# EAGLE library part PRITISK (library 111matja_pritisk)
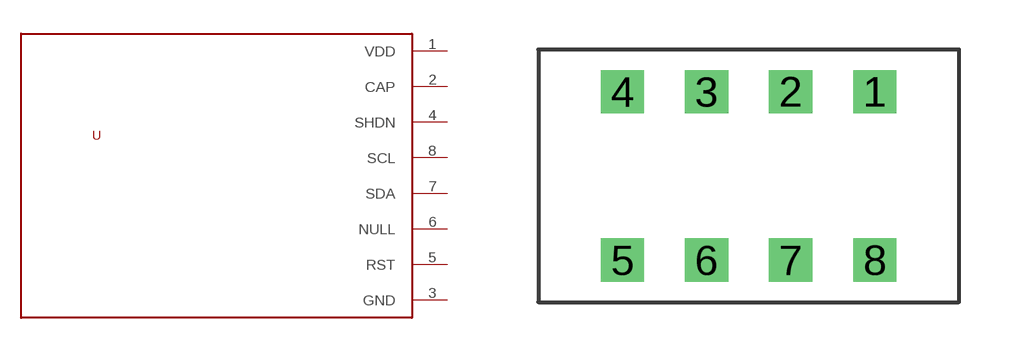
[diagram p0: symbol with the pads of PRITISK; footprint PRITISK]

Designator prefix -

## PRITISK  [PRITISK]
1  VDD
2  CAP
3  GND
4  SHDN
5  RST
6  NULL
7  SDA
8  SCL

## Footprint PRITISK (pad centres in mm)
drill 0.8 square: 1 3.81,2.54; 2 1.27,2.54; 3 -1.27,2.54; 4 -3.81,2.54; 5 -3.81,-2.54; 6 -1.27,-2.54; 7 1.27,-2.54; 8 3.81,-2.54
